PROGRAM MAIN_CM
VAR CONSTANT
	cInitFFT		: ST_CM_RealFFT_InitPars := ( 	nFFT_Length 		:= cFFTLength, 
													bHalfSpec 			:= TRUE, 
													bForward 			:= TRUE );
													
	cInitZoomFFT 	: ST_CM_ZoomFFT_InitPars := (	nFFT_Length 		:= cFFTLength,
													fSampleRate			:= cSampleRate,
													fCenter				:= cSetFrequency,
													nDecimationFactor	:= cDecimationFactor);															
END_VAR

VAR		
	fbFFT				: FB_CMA_RealFFT := ( stInitPars := cInitFFT, nOwnID := eID_FFT, aDestIDs := [eID_SinkFFT] );										
	fbZoomFFT			: FB_CMA_ZoomFFT := ( stInitPars := cInitZoomFFT, nOwnID := eID_ZoomFFT, aDestIDs := [eID_SinkZoomFFT] );

	(* error monitoring *)
	fbErrHist	: FB_HRErrHist;												
END_VAR

// Call FFT 
fbFFT.Call();
IF fbFFT.bError THEN
	fbErrHist.AddError(bErr:=TRUE, hrErrCode:=fbFFT.hrErrorCode, sErrSource:='MAIN_CM.fbFFT'); // error monitoring
	// ToDo: if error
END_IF

// Call ZoomFFT 
fbZoomFFT.Call();
IF fbZoomFFT.bError THEN
	fbErrHist.AddError(bErr:=TRUE, hrErrCode:=fbZoomFFT.hrErrorCode, sErrSource:='MAIN_CM.fbZoomFFT'); // error monitoring
	// ToDo: if error
END_IF

END_PROGRAM
